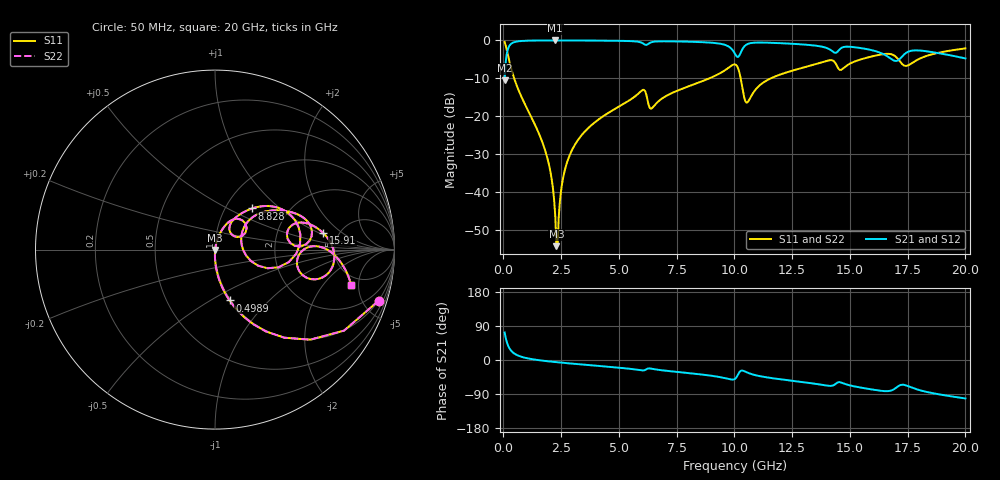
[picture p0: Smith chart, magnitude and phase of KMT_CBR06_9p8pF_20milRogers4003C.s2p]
! Data measured by Modelithics Inc. support@modelithics.com 813-866-6335
! KEMET CBR0603 9.8pF, Pad Width= 0.851mm, Pad Length= 0.64mm, Pad Gap= 0.62mm, 20mil Rogers 4003C substrate Data, January 2022
# hz S ma R 50
! 2 Port Network Data from SP1.SP block
! freq  magS11  angS11  magS21  angS21  magS12  angS12  magS22  angS22
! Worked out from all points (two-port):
!   401 points, 50 MHz to 20 GHz, reference 50 ohm
!   highest |S21| = -0.01 dB at 2.244 GHz (marker M1); lowest = -10.6 dB at 50 MHz (marker M2)
!   |S21| within 3 dB of the highest: 163.1 MHz to 9.973 GHz (9.81 GHz wide, 194 % of centre); 10.29 GHz to 14.28 GHz (3.989 GHz wide, 32.5 % of centre)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
!   lowest |S11| = -54.2 dB at 2.294 GHz (marker M3), VSWR 1.00, Z = 50.1 - j0.163 ohm
!   |S11| at or under -10 dB: 464.3 MHz to 8.911 GHz (8.447 GHz wide, 180 % of centre); 10.27 GHz to 11.57 GHz (1.304 GHz wide, 11.9 % of centre)
!   |S22| runs from -54.2 to -0.4 dB; largest |S21 - S12| = 0
!   S11 on the Smith chart (normalised r, x): 50 MHz: 0.99, -6.39; 498.9 MHz: 0.99, -0.61; 8.828 GHz: 1.33, +0.67; 15.91 GHz: 3.80, +1.10; 20 GHz: 3.96, -4.07
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5e7  0.9549 -17.4  0.2965 72.6  0.2965 72.6  0.9549 -17.4
2.99375e8  0.4675 -62.8  0.8833 27.1  0.8833 27.1  0.4675 -62.8
4.98875e8  0.2944 -74.0  0.955 15.9  0.955 15.9  0.2944 -74.0
1.8455e9  0.03243 -90.8  0.9983 -2.8  0.9983 -2.8  0.03243 -90.8
2.094875e9  0.01444 -89.8  0.9986 -4.5  0.9986 -4.5  0.01444 -89.8
2.2445e9  0.004787 -80.7  0.9987 -5.4  0.9987 -5.4  0.004787 -80.7
2.294375e9  0.001949 -56.8  0.9987 -5.7  0.9987 -5.7  0.001949 -56.8
2.693375e9  0.02154 78.4  0.9984 -8.0  0.9984 -8.0  0.02154 78.4
3.391625e9  0.05681 76.7  0.9968 -11.8  0.9968 -11.8  0.05681 76.7
5.985125e9  0.2183 50.8  0.932 -27.4  0.932 -27.4  0.2183 50.8
6.384125e9  0.1256 42.7  0.9408 -22.6  0.9408 -22.6  0.1256 42.7
6.73325e9  0.16 58.6  0.9723 -26.1  0.9723 -26.1  0.16 58.6
8.828e9  0.3086 47.9  0.9406 -40.2  0.9406 -40.2  0.3086 47.9
1.0025e10  0.4832 10.0  0.6658 -49.9  0.6658 -49.9  0.4832 10.0
1.027438e10  0.311 -19.5  0.6913 -28.6  0.6913 -28.6  0.311 -19.5
1.057362e10  0.1538 18.1  0.8968 -33.4  0.8968 -33.4  0.1538 18.1
1.14215e10  0.2996 40.1  0.9336 -46.0  0.9336 -46.0  0.2996 40.1
1.336662e10  0.4728 26.2  0.863 -61.7  0.863 -61.7  0.4728 26.2
1.591025e10  0.6109 8.6  0.7485 -77.3  0.7485 -77.3  0.6109 8.6
1.670825e10  0.6648 -6.8  0.5929 -81.7  0.5929 -81.7  0.6648 -6.8
1.74065e10  0.4614 -8.4  0.6759 -66.6  0.6759 -66.6  0.4614 -8.4
2e10  0.7842 -14.6  0.5787 -101.5  0.5787 -101.5  0.7842 -14.6
